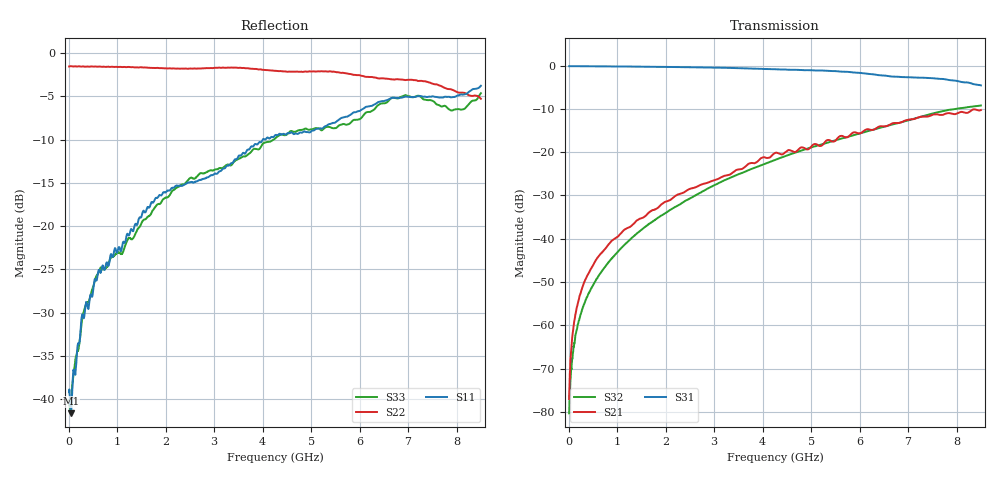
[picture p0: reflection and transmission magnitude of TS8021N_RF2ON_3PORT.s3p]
!Created with skrf (http://scikit-rf.org).
# GHz S RI R 50.0
!freq ReS11 ImS11 ReS12 ImS12 ReS13 ImS13
! ReS21 ImS21 ReS22 ImS22 ReS23 ImS23
! ReS31 ImS31 ReS32 ImS32 ReS33 ImS33
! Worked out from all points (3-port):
!   1601 points, 10 MHz to 8.5 GHz, reference 50 ohm
!   strongest paths, dB at 10 MHz, 2.132 GHz, 4.255 GHz, 6.378 GHz, 8.5 GHz:
!     S31: -0.1, -0.3, -0.9, -2.2, -4.6
!     S21: -77.0, -30.7, -20.2, -14.2, -10.3
!     S32: -80.3, -33.1, -21.8, -14.5, -9.2
!   lowest |S11| = -41.6 dB at 47.14 MHz (marker M1), VSWR 1.02, Z = 50.7 - j0.483 ohm
!   |S11| at or under -10 dB: start of sweep to 4.003 GHz; 4.046363 GHz to 4.051834 GHz (5.471 MHz wide, 0.135 % of centre)
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0.01  0.011 0.000261  9.29e-05 0.000105  0.9848 -0.00308
      8.78e-05 0.000111  -0.8363 0.00313  9.47e-05 5.57e-05
      0.9846 -0.00307  8.75e-05 4.01e-05  0.0098 0.000503
0.04714375  0.00678 -0.00476  8.26e-05 0.000461  0.985 -0.0136
            9.28e-05 0.000461  -0.8396 0.0109  8.5e-05 0.000251
            0.9849 -0.0133  9.47e-05 0.00026  0.00833 -0.0037
0.1267375  0.0062 -0.0127  7.51e-05 0.00121  0.9837 -0.0354
           8.03e-05 0.00121  -0.8382 0.027  5.77e-05 0.000689
           0.9835 -0.0355  7.01e-05 0.000664  0.0086 -0.0134
0.285925  0.00529 -0.0302  -6.2e-05 0.00278  0.9796 -0.0799
          -8.44e-05 0.00276  -0.835 0.0598  -0.000128 0.00155
          0.9797 -0.08  -0.000112 0.00156  0.00685 -0.0291
0.8696125  -0.0109 -0.0679  -0.00109 0.0092  0.949 -0.2355
           -0.00109 0.00914  -0.8101 0.1912  -0.00159 0.00548
           0.949 -0.2354  -0.00159 0.00553  -0.00927 -0.0651
2.143112  -0.0677 -0.1523  -0.00397 0.0291  0.7945 -0.544
          -0.00397 0.0292  -0.6942 0.427  -0.00498 0.0218
          0.7952 -0.5442  -0.00496 0.0218  -0.0947 -0.1296
4.255  -0.2971 -0.154  0.0247 0.0947  0.3239 -0.8467
       0.0246 0.0946  -0.3324 0.7159  0.0217 0.0784
       0.3226 -0.846  0.0218 0.0785  -0.3106 -0.0776
6.977106  -0.5124 0.2248  0.2066 0.1136  -0.2898 -0.673
          0.206 0.1136  0.2902 0.6361  0.2183 0.0742
          -0.2893 -0.6737  0.2188 0.074  -0.4741 0.3112
7.8208  -0.3372 0.4449  0.2789 0.0476  -0.4166 -0.5449
        0.2784 0.0478  0.383 0.4871  0.3064 -0.00678
        -0.4175 -0.5439  0.3068 -0.00728  -0.331 0.3448
8.5  -0.3158 0.5643  0.3061 0.00496  -0.4532 -0.3785
     0.3064 0.00475  0.4428 0.3166  0.3286 -0.1103
     -0.4534 -0.3786  0.3283 -0.1101  -0.1414 0.5686
